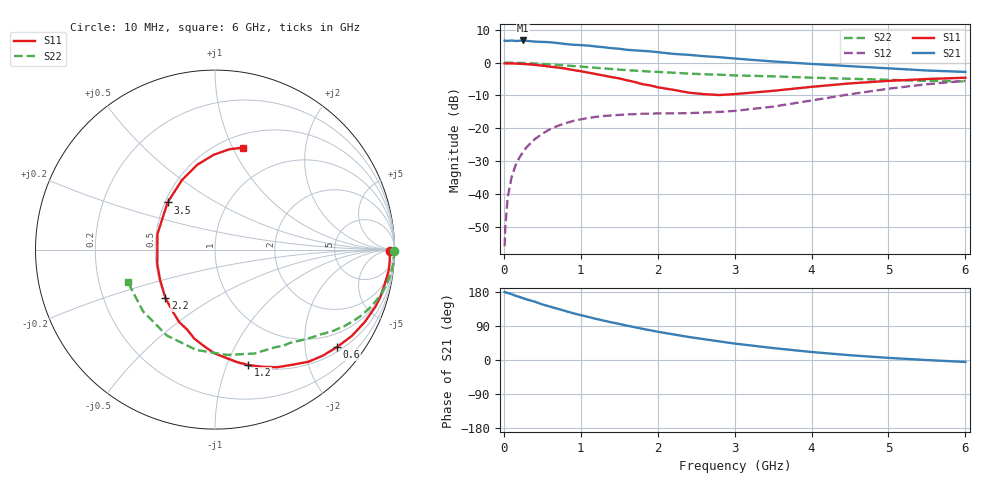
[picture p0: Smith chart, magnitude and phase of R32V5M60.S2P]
! SIEMENS Small Signal Semiconductors
! BFR181
! Si NPN RF Bipolar Junction Transistor in SOT23
! VCE = 2.5 V  IC = 0.6 mA
! Common Emitter S-Parameters:  May  1996
# GHz  S  MA  R  50
!  f  S11  S21  S12  S22
! GHz  MAG  ANG  MAG  ANG  MAG  ANG  MAG  ANG
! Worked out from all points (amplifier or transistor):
!   36 points, 10 MHz to 6 GHz, reference 50 ohm
!   highest |S21| = 6.8 dB at 250 MHz (marker M1)
!   |S21| within 3 dB of that: start of sweep to 1.693 GHz
!   unconditionally stable (mu >= 1): 2.261 GHz to 3.878 GHz
!   at 250 MHz: K = 0.13, MSG = 17.0 dB, |S12| = -27.2 dB
!   at 1.4 GHz: K = 0.65, MSG = 10.2 dB, |S12| = -16.1 dB
!   at 6 GHz: K = 0.91, MSG = 1.4 dB, |S12| = -5.5 dB
!   S11 on the Smith chart (normalised r, x): 10 MHz: 71, -32; 600 MHz: 0.61, -2.73; 1.2 GHz: 0.51, -1.19; 2.2 GHz: 0.50, -0.32; 3.5 GHz: 0.52, +0.31; 6 GHz: 0.63, +1.10
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0.01  0.9768 -0.6  2.174 179.7  0.0016 89.7  0.9998 -0.3
0.02  0.9739 -1.3  2.15 178.5  0.0032 86.3  0.9996 -0.7
0.05  0.9755 -3.2  2.15 176.9  0.0088 88.6  0.9985 -1.5
0.1  0.9752 -6.5  2.18 173.8  0.0178 86.3  0.9968 -3.0
0.15  0.9688 -9.6  2.142 169.7  0.0269 82.8  0.995 -4.7
0.25  0.9575 -16.3  2.181 163.2  0.0436 78.3  0.9888 -7.7
0.4  0.9271 -25.7  2.095 154.1  0.0679 72.4  0.9731 -12.0
0.5  0.9014 -32.3  2.073 146.7  0.0828 68.2  0.9594 -14.9
0.6  0.8698 -38.6  2.051 140.9  0.0968 64.3  0.9419 -17.6
0.8  0.8133 -50.2  1.927 129.3  0.1194 57.1  0.9065 -22.5
1.1  0.7043 -68.0  1.82 113.5  0.1439 48.4  0.8528 -28.8
1.2  0.6686 -74.0  1.764 108.4  0.1495 45.9  0.8351 -30.9
1.4  0.6027 -84.8  1.664 99.2  0.1571 41.8  0.8004 -34.4
1.8  0.471 -109.3  1.514 82.4  0.167 37.2  0.7457 -39.9
2.2  0.3863 -135.6  1.363 67.7  0.1688 36.2  0.7025 -45.7
2.4  0.3498 -151.0  1.318 60.9  0.17 37.3  0.6828 -48.5
2.8  0.3214 178.6  1.213 49.2  0.1779 40.7  0.6564 -54.8
3.5  0.3725 135.2  1.044 31.5  0.2139 48.3  0.6191 -69.3
4.5  0.4834 101.7  0.884 12.6  0.3304 48.8  0.5688 -100.5
5  0.5278 90.9  0.82 5.6  0.4012 43.6  0.5488 -119.3
5.5  0.5638 82.1  0.76 -0.2  0.4697 36.1  0.5282 -139.5
6  0.5898 74.5  0.723 -5.2  0.5292 27.6  0.5185 -159.9
